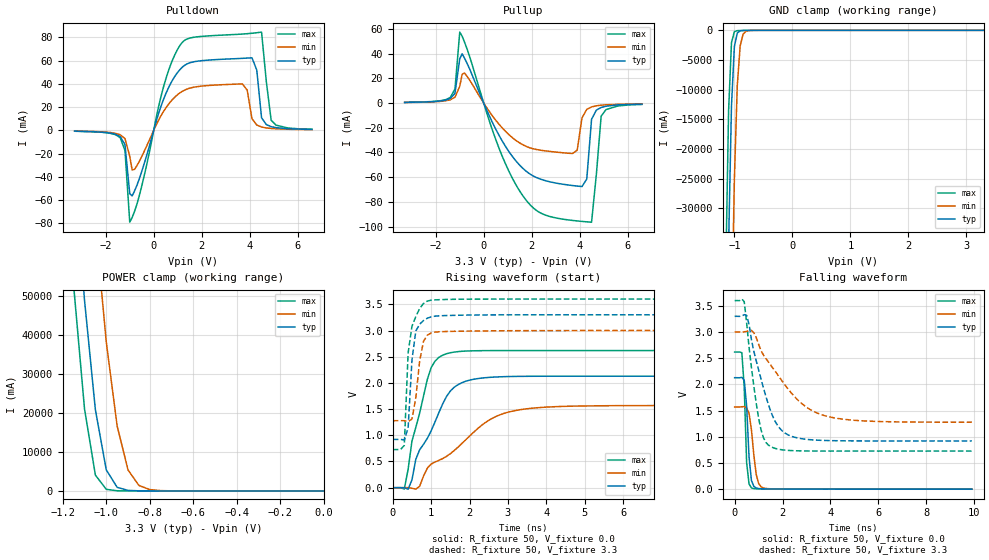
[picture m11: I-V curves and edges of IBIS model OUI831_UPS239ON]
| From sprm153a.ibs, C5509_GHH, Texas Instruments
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| Pin_model   OUI831_UPS239ON
[Model]   OUI831_UPS239ON
 Model_type   I/O
 Polarity   Non-Inverting
 Enable   Active-Low
 Vinl  =  1.08
 Vinh  =  2.1
 Vmeas =  1.5
|Variable   typ   min   max
 C_comp   2.349pF   2.328pF   2.418pF
[Add Submodel]
| Submodel_name   Mode
UPS239BH   Non-Driving
[Temperature Range]   25   125   -40
[Voltage Range]   3.3   3   3.6
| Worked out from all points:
|   slope of the pulldown table from 0 to 0.495 V, typ, clamps not added: 16 ohm
|   slope of the pullup table from 0 to 0.495 V, typ, clamps not added: 23.8 ohm
|   GND clamp passes 1 mA (typ) near -0.59 V on its own axis
|   POWER clamp passes 1 mA (typ) near -0.70 V on its own axis
|   rising waveform, R_fixture 50, V_fixture 0.0: 20-80 % time 803ps typ, 1.58ns min, 481ps max; typ from 0 V to 2.13 V
|   rising waveform, R_fixture 50, V_fixture 3.3: 20-80 % time 150ps typ, 186ps min, 161ps max; typ from 0.921 V to 3.3 V
|   falling waveform, R_fixture 50, V_fixture 0.0: 20-80 % time 166ps typ, 229ps min, 121ps max; typ from 2.13 V to 0 V
|   falling waveform, R_fixture 50, V_fixture 3.3: 20-80 % time 870ps typ, 1.74ns min, 491ps max; typ from 3.3 V to 0.921 V
[GND Clamp]
|Voltage   I(typ)   I(min)   I(max)
-3.3V     -2.131kA   -2.172kA   -2.112kA
-1.15V    -69.25A    -121A      -41.3A
-1.1V     -36.04A    -83.7A     -13.64A
-1.05V    -12.77A    -50.83A    -2.067A
-1V       -2.726A    -25.08A    -235.7mA
-950mV    -452.8mA   -9.272A    -58.81mA
-900mV    -87.46mA   -2.634A    -35.31mA
-850mV    -28.98mA   -661.7mA   -25.36mA
-800mV    -15.75mA   -165.5mA   -17.4mA
-600mV    -1.159mA   -2.526mA   -779.5uA
3.3V      227.8pA    2.608nA    193.2pA
[POWER Clamp]
|Voltage   I(typ)   I(min)   I(max)
-3.3V     2.152kA    2.199kA    2.128kA
-1.15V    84.65A     142.8A     52.53A
-1.1V     48.8A      103.8A     20.98A
-1.05V    20.76A     68.2A      4.051A
-1V       5.397A     38.14A     409.1mA
-950mV    921.2mA    16.63A     39.37mA
-900mV    138.6mA    5.377A     6.944mA
-850mV    22.05mA    1.408A     3.344mA
-800mV    4.684mA    339.9mA    2.327mA
-750mV    1.724mA    80.96mA    1.635mA
0V        0A         0A         0A
[Pulldown]
|Voltage   I(typ)   I(min)   I(max)
-3.3V     -700uA     -600uA     -800uA
-1.4V     -5.36mA    -3.81mA    -6.26mA
-1.2V     -12.24mA   -7.11mA    -17.31mA
-1V       -54.58mA   -22.44mA   -78.99mA
-800mV    -52.16mA   -33.54mA   -69.68mA
400mV     26.07mA    15.89mA    36.64mA
1.1V      52.31mA    32.25mA    73.11mA
3.7V      61.86mA    39.87mA    82.75mA
4.1V      62.32mA    9.97mA     83.41mA
4.5V      10.73mA    2.83mA     84.43mA
4.9V      3.13mA     1.59mA     8.65mA
6.6V      700uA      600uA      1mA
[Pullup]
|Voltage   I(typ)   I(min)   I(max)
-3.3V     500uA      500uA      600uA
-1.4V     3.68mA     2.66mA     4.45mA
-1.2V     7.9mA      4.73mA     11.41mA
-1V       35.94mA    13.64mA    57.52mA
850mV     -33.18mA   -21.68mA   -46.54mA
2.15V     -59.85mA   -37.37mA   -86.19mA
3.7V      -66.75mA   -40.84mA   -95.02mA
4.1V      -67.58mA   -12.01mA   -95.82mA
4.3V      -61.52mA   -5.05mA    -96.15mA
4.5V      -13.11mA   -3.07mA    -96.45mA
4.9V      -3.54mA    -1.69mA    -10.6mA
6.6V      -800uA     -600uA     -1.1mA
[Ramp]
|Variable   typ   min   max
 dV/dt_r   1.29V/0.810ns   0.95V/1.590ns   1.59V/0.490ns
 dV/dt_f   1.43V/0.870ns   1.03V/1.740ns   1.72V/0.490ns
 R_load =  50
[Rising Waveform]
 R_fixture =   50
 V_fixture =   0.0
 V_fixture_min =  0.0
 V_fixture_max =  0.0
|Time   V(typ)   V(min)   V(max)
0s        8.607nV    2.953uV    10.28nV
300ps     -531.3uV   1.3mV      -26.87mV
500ps     149.5mV    -11.43mV   890.3mV
700ps     723mV      27.06mV    1.423V
900ps     941.5mV    373.3mV    2.065V
1.1ns     1.254V     490.1mV    2.415V
1.4ns     1.74V      598.1mV    2.557V
2ns       2.052V     984.4mV    2.61V
3.3ns     2.125V     1.486V     2.617V
9.9ns     2.128V     1.569V     2.617V
[Rising Waveform]
 R_fixture =   50
 V_fixture =   3.3
 V_fixture_min =  3
 V_fixture_max =  3.6
|Time   V(typ)   V(min)   V(max)
0s        920.7mV    1.278V     727mV
300ps     910.9mV    1.278V     805.6mV
400ps     1.141V     1.262V     2.571V
500ps     2.439V     1.311V     3.081V
600ps     2.99V      1.715V     3.265V
700ps     3.12V      2.417V     3.419V
800ps     3.189V     2.793V     3.515V
900ps     3.234V     2.911V     3.562V
1.8ns     3.292V     2.987V     3.597V
9.9ns     3.3V       3V         3.6V
[Falling Waveform]
 R_fixture =   50
 V_fixture =   0.0
 V_fixture_min =  0.0
 V_fixture_max =  0.0
|Time   V(typ)   V(min)   V(max)
0s        2.128V     1.569V     2.617V
300ps     2.135V     1.573V     2.606V
400ps     2.079V     1.577V     1.948V
500ps     1.591V     1.55V      511.3mV
600ps     619.7mV    1.449V     101.9mV
700ps     167.2mV    1.141V     23.71mV
900ps     21.65mV    282.3mV    7.575mV
1ns       11.4mV     109.8mV    6.062mV
1.2ns     6.451mV    23.29mV    4.123mV
9.9ns     -102.8nV   1.766uV    22.89nV
[Falling Waveform]
 R_fixture =   50
 V_fixture =   3.3
 V_fixture_min =  3
 V_fixture_max =  3.6
|Time   V(typ)   V(min)   V(max)
0s        3.3V       3V         3.6V
400ps     3.331V     3.003V     3.58V
600ps     3.149V     3.027V     2.716V
1ns       2.278V     2.766V     1.355V
1.2ns     1.938V     2.562V     986mV
1.5ns     1.495V     2.372V     814mV
2.2ns     1.044V     1.93V      741.1mV
3ns       951.1mV    1.565V     728.9mV
3.8ns     929mV      1.398V     727mV
9.9ns     920.7mV    1.278V     727mV
